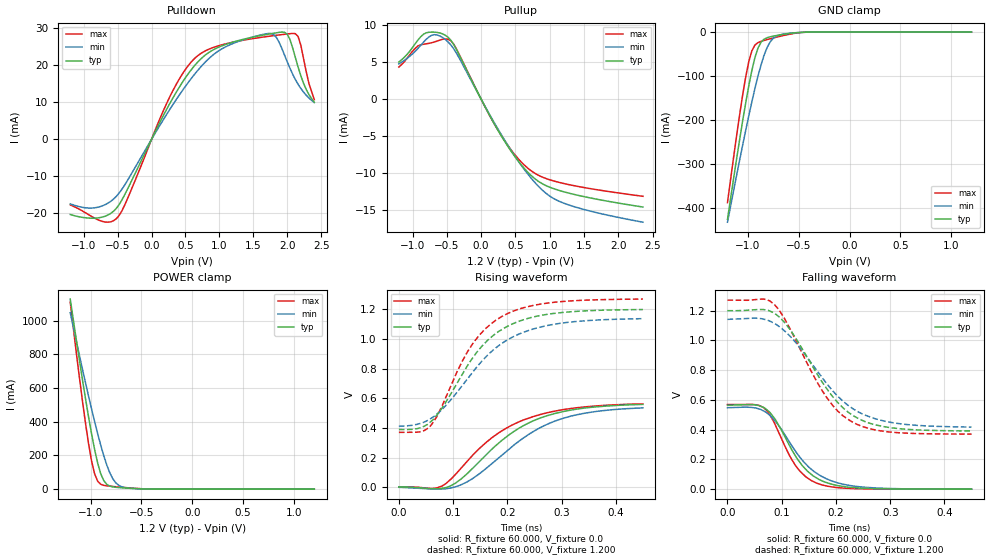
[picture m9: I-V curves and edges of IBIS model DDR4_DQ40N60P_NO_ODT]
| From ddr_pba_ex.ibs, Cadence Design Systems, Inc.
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|   Model DDR4_DQ40N60P_NO_ODT
[Model]   DDR4_DQ40N60P_NO_ODT
Model_type I/O
Polarity   Non-Inverting
Enable   Active-High
Vinl   =   0.823V
Vinh   =   0.887V
C_comp   1.715pF   1.731pF   1.724pF
C_comp_pullup   0.538pF   0.595pF   0.525pF
C_comp_pulldown 1.177pF   1.135pF   1.198pF
[Model Spec]
Vinh   0.887V   NA   NA
Vinl   0.823V   NA   NA
Vmeas   0.840V   NA   NA
[Temperature Range]   27.000   0.125k   -40.000
[Voltage Range]   1.200V   1.140V   1.270V
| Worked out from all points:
|   slope of the pulldown table from 0 to 0.18 V, typ, clamps not added: 27.2 ohm
|   slope of the pullup table from 0 to 0.18 V, typ, clamps not added: 57.4 ohm
|   GND clamp passes 1 mA (typ) near -0.50 V on its own axis
|   POWER clamp passes 1 mA (typ) near -0.46 V on its own axis
|   rising waveform, R_fixture 60.000, V_fixture 0.0: 20-80 % time 115ps typ, 121ps min, 116ps max; typ from 0.001 V to 0.558 V
|   rising waveform, R_fixture 60.000, V_fixture 1.200: 20-80 % time 95.9ps typ, 111ps min, 86ps max; typ from 0.389 V to 1.2 V
|   falling waveform, R_fixture 60.000, V_fixture 0.0: 20-80 % time 59.2ps typ, 70.8ps min, 50.4ps max; typ from 0.565 V to 0 V
|   falling waveform, R_fixture 60.000, V_fixture 1.200: 20-80 % time 89.3ps typ, 99.6ps min, 83.4ps max; typ from 1.2 V to 0.391 V
[Pulldown]
|Voltage   I(typ)   I(min)   I(max)
-1.2V     -20.33mA   -17.47mA   -17.73mA
-840mV    -21.33mA   -18.52mA   -21.33mA
-520mV    -18.67mA   -15.43mA   -21.47mA
400mV     13.8mA     11.7mA     16mA
640mV     20.01mA    17.69mA    21.92mA
960mV     24.62mA    23.51mA    25.09mA
1.76V     28.51mA    28.56mA    27.88mA
1.84V     28.75mA    27.53mA    28.07mA
2V        28.39mA    20.97mA    28.43mA
2.12V     22.12mA    16.15mA    28.51mA
2.2V      17.21mA    13.75mA    25.48mA
2.4V      9.967mA    9.905mA    10.69mA
[Pullup]
|Voltage   I(typ)   I(min)   I(max)
-1.2V     5.02mA     4.773mA    4.338mA
-960mV    7.516mA    6.485mA    6.876mA
-840mV    8.783mA    7.706mA    7.425mA
-720mV    9.066mA    8.641mA    7.63mA
-560mV    8.818mA    8.321mA    8.099mA
-400mV    7.394mA    6.807mA    7.432mA
280mV     -4.745mA   -4.576mA   -4.71mA
520mV     -8.111mA   -8.075mA   -7.827mA
760mV     -10.57mA   -11.01mA   -9.882mA
960mV     -11.75mA   -12.82mA   -10.77mA
1.2V      -12.51mA   -14.04mA   -11.39mA
2.36V     -14.59mA   -16.63mA   -13.13mA
[GND_clamp]
|Voltage   I(typ)   I(min)   I(max)
-1.2V     -426.2mA   -432.8mA   -388.3mA
-1.08V    -244.1mA   -290.9mA   -187.6mA
-1.02V    -160.2mA   -222.9mA   -101.2mA
-990mV    -121.8mA   -190.1mA   -66.76mA
-960mV    -87.12mA   -158.5mA   -42.47mA
-900mV    -36.37mA   -100.2mA   -23.99mA
-840mV    -16.17mA   -52.6mA    -18.98mA
-810mV    -12.75mA   -34.94mA   -17.06mA
-750mV    -9.219mA   -14.09mA   -13.42mA
-600mV    -3.476mA   -2.979mA   -5.372mA
-390mV    -77.95uA   -145.6uA   -88.64uA
1.2V      1.573nA    185.8nA    251.5pA
[POWER_clamp]
|Voltage   I(typ)   I(min)   I(max)
-1.2V     1.129A     1.047A     1.109A
-1.08V    651.1mA    713.3mA    524.8mA
-1.02V    430.1mA    553.1mA    270.8mA
-990mV    328mA      475.7mA    167mA
-960mV    234.7mA    400.6mA    90.32mA
-930mV    154.2mA    328.7mA    47.17mA
-900mV    91.53mA    260.8mA    29.3mA
-840mV    28.2mA     142.5mA    19.67mA
-780mV    13.3mA     60.49mA    15.94mA
-720mV    9.309mA    21.57mA    12.7mA
-660mV    6.902mA    8.818mA    9.642mA
1.2V      -4.11nA    -153.5nA   -872pA
[Ramp]
| variable   typ   min   max
dV/dt_r 0.301/0.112n   0.290/0.122n   0.299/0.111n
dV/dt_f 0.453/91.493p   0.403/0.102n   0.505/85.674p
R_load = 50.000
| The next line is not an IBIS keyword
| [Initial Delay]   0.325ns   0.535ns   0.200ns
[Rising Waveform]
R_fixture= 60.000
V_fixture= 0.0
V_fixture_min= 0.0
V_fixture_max= 0.0
|time   V(typ)   V(min)   V(max)
0s        1.44mV     -740.2uV   336.8uV
69ps      -10.7mV    -13.14mV   -5.941mV
94ps      6.685mV    -6.851mV   47.68mV
124ps     84.39mV    31.91mV    166.9mV
168ps     244.1mV    147.9mV    323.5mV
199ps     341.9mV    244.5mV    399.9mV
238ps     430.9mV    352.5mV    464.1mV
281ps     490.1mV    436.1mV    508mV
322ps     522.9mV    483.6mV    532.9mV
450ps     558.2mV    534.6mV    562.1mV
[Rising Waveform]
R_fixture= 60.000
V_fixture= 1.200
V_fixture_min= 1.140
V_fixture_max= 1.270
|time   V(typ)   V(min)   V(max)
0s        389mV      411.3mV    369.5mV
38ps      399mV      428.2mV    372.4mV
60ps      445.3mV    465.3mV    420.4mV
83ps      551.6mV    536.6mV    575.7mV
127ps     821.9mV    732.6mV    915.9mV
158ps     969.5mV    869.4mV    1.063V
189ps     1.061V     967.2mV    1.149V
224ps     1.122V     1.037V     1.204V
282ps     1.17V      1.096V     1.245V
450ps     1.198V     1.136V     1.268V
[Falling Waveform]
R_fixture= 60.000
V_fixture= 0.0
V_fixture_min= 0.0
V_fixture_max= 0.0
|time   V(typ)   V(min)   V(max)
0s        564.7mV    547.3mV    569mV
54ps      564.5mV    543.3mV    566.4mV
71ps      538mV      517.1mV    533.3mV
88ps      469.5mV    458.2mV    433.2mV
124ps     231.3mV    262.6mV    165.5mV
148ps     119.2mV    155mV      73.95mV
173ps     57.98mV    87.27mV    29.68mV
202ps     25.03mV    43.52mV    10.65mV
251ps     6.091mV    13.44mV    2.225mV
450ps     162.1uV    201.7uV    72.77uV
[Falling Waveform]
R_fixture= 60.000
V_fixture= 1.200
V_fixture_min= 1.140
V_fixture_max= 1.270
|time   V(typ)   V(min)   V(max)
0s        1.199V     1.141V     1.27V
66ps      1.207V     1.143V     1.277V
86ps      1.183V     1.114V     1.243V
115ps     1.075V     1.029V     1.08V
182ps     680.2mV    713.1mV    620.3mV
203ps     583.1mV    625.6mV    525.9mV
228ps     503.4mV    548.7mV    456mV
261ps     444.3mV    487.4mV    407.4mV
301ps     412.9mV    448.8mV    383.4mV
450ps     391.2mV    417mV      369.9mV
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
